| TEXAS INSTRUMENTS INCORPORATED
| Standard Linear and Logic Group
| IBIS Model of PCA9544A
| 4-CHANNEL I2C AND SMBus MULTIPLEXER WITH INTERRUPT LOGIC
| This file contains package information for the following:
|  TSSOP 20-pin (PW) package as [Component] PCA9544_PW
|  QFN 20-pin (RGY) package as [Component] PCA9544_RGY
|  SOIC 20-pin (DW) package as [Component] PCA9544_DW
|  TVSOP 20-pin (DGV) package as [Component] PCA9544_DGV
|  VFBGA 20-pin (GQN) package as [Component] PCA9544_GQN
|  VFBGA 20-pin (ZQN) package as [Component] PCA9544_ZQN
| This device can be powered at the following Vccs:
|  5 volt Vcc
|  3.3 volt Vcc
|  2.5 volt Vcc
| This file provides unique models under the [Model Selector] for each Vcc.
| For operation at a specific Vcc, select the appropriate model after each
| [Model Selector] keyword.
[IBIS Ver]   3.2
[Comment char]  |_char
[File Name]   pca9544a.ibs
[File Rev]   1.1 | a_die
[Date]   February 12, 2007
[Source]   Data created from TI-SPICE simulations at TI-SLL.
[Notes]   The following is an IBIS list for the PCA9544A.
   Please contact sllibis@ti.com with questions and
   comments concerning SLL IBIS models.
   This IBIS model is created from a BA (back annotated netlist)
   - FILE REV HISTORY
   - 1.1 Release IBIS file on 2/13/07
   - Power clamp data has been deleted in all models except
   SDA terminator models as there is no power-clamp diode.
   - Non-monotonic data due to FET characteristics.
[Disclaimer] Property of Texas Instruments Incorporated.  Unauthorized
   reproduction and/or distribution is strictly prohibited.
   This product is protected under copyright law.
   Created  2007, (C) Copyright  2007, Texas Instruments
   Incorporated, All Rights Reserved
   UNLESS THERE IS A SIGNED, WRITTEN AGREEMENT TO THE
   CONTRARY, TEXAS INSTRUMENTS (TI) IS PROVIDING THE IBIS
   MODELS  AND WITHOUT ANY WARRANTY, EXPRESSED OR
   IMPLIED.  TI assumes no liability for:
   1) the accuracy of the IBIS models provided to your
   company;
   2) the proper functioning of these IBIS Models in your
   design or for any resulting applications; or
   3) infringement of patents, copyrights or intellectual
   property rights resulting from your use of these IBIS
   models.
   TI provides IBIS Models as a service to our customers.
   You and your company shall not distribute, sell or give
   these models to anyone else without prior written
   permission from TI.
   TI reserves the right to make changes to our products or
   to discontinue any semiconductor product or service
   without notice, and advises our customers to obtain the
   latest version of relevant information to verify, before
   placing orders, that the information being relied on is
   current.
   Please be aware that your receipt and use of the IBIS
   information provided shall serve as acceptance of these
   terms and conditions.  If you do not accept these terms,
   you should return or destroy the IBIS models and any
   other accompanying information immediately.
| Component PCA9544A_PW 20-PIN TSSOP
[Component]   PCA9544A_PW
[Manufacturer]   Texas Instruments, Inc.
[Package]
|   typ   min   max
R_pkg   5.000e-02   4.200e-02   6.000e-02
L_pkg   2.802e-09   2.248e-09   3.553e-09
C_pkg   3.170e-13   2.020e-13   4.430e-13
[Pin]   signal_name   model_name   R_pin   L_pin   C_pin
1   A0   PCA9544_A   5.500e-02   3.461e-09   4.400e-13
2   A1   PCA9544_A   5.500e-02   3.150e-09   4.010e-13
3   A2   PCA9544_A   4.200e-02   2.619e-09   3.020e-13
4   NINT0   PCA9544_INTX   4.500e-02   2.273e-09   2.020e-13
5   SD0   PCA9544_SDX   4.500e-02   2.248e-09   2.240e-13
6   SC0   PCA9544_SCX   4.500e-02   2.273e-09   2.260e-13
7   NINT1   PCA9544_INTX   4.400e-02   2.323e-09   2.050e-13
8   SD1   PCA9544_SDX   4.600e-02   2.704e-09   3.070e-13
9   SC1   PCA9544_SCX   6.000e-02   3.265e-09   4.110e-13
10   GND   GND   5.700e-02   3.506e-09   4.360e-13
11   NINT2   PCA9544_INTX   5.800e-02   3.553e-09   4.370e-13
12   SD2   PCA9544_SDX   5.800e-02   3.193e-09   4.050e-13
13   SC2   PCA9544_SCX   4.200e-02   2.704e-09   3.110e-13
14   NINT3   PCA9544_INTX   4.600e-02   2.392e-09   2.100e-13
15   SD3   PCA9544_SDX   4.700e-02   2.334e-09   2.290e-13
16   SC3   PCA9544_SCX   4.700e-02   2.300e-09   2.270e-13
17   NINT   PCA9544_INT   4.700e-02   2.349e-09   2.070e-13
18   SCL   PCA9544_SCL   4.500e-02   2.677e-09   3.060e-13
19   SDA   PCA9544_SDA   6.000e-02   3.235e-09   4.060e-13
20   VCC   POWER   5.600e-02   3.487e-09   4.430e-13
| Component PCA9544A_RGY 20-PIN QFN
[Component]   PCA9544A_RGY
[Manufacturer]   Texas Instruments, Inc.
[Package]
|   typ   min   max
R_pkg   5.000e-02   4.600e-02   5.500e-02
L_pkg   1.119e-09   1.025e-09   1.227e-09
C_pkg   3.520e-13   3.440e-13   3.630e-13
[Pin]   signal_name   model_name   R_pin   L_pin   C_pin
1   A0   PCA9544_A   5.200e-02   1.167e-09   3.600e-13
2   A1   PCA9544_A   4.700e-02   1.049e-09   3.440e-13
3   A2   PCA9544_A   4.700e-02   1.055e-09   3.450e-13
4   NINT0   PCA9544_INTX   5.000e-02   1.119e-09   3.500e-13
5   SD0   PCA9544_SDX   5.500e-02   1.227e-09   3.600e-13
6   SC0   PCA9544_SCX   5.200e-02   1.167e-09   3.550e-13
7   NINT1   PCA9544_INTX   4.900e-02   1.087e-09   3.480e-13
8   SD1   PCA9544_SDX   4.700e-02   1.054e-09   3.460e-13
9   SC1   PCA9544_SCX   4.900e-02   1.091e-09   3.490e-13
10   GND   GND   5.300e-02   1.184e-09   3.620e-13
11   NINT2   PCA9544_INTX   5.300e-02   1.181e-09   3.600e-13
12   SD2   PCA9544_SDX   5.000e-02   1.108e-09   3.490e-13
13   SC2   PCA9544_SCX   4.800e-02   1.075e-09   3.470e-13
14   NINT3   PCA9544_INTX   5.000e-02   1.107e-09   3.490e-13
15   SD3   PCA9544_SDX   5.400e-02   1.200e-09   3.620e-13
16   SC3   PCA9544_SCX   5.100e-02   1.141e-09   3.570e-13
17   NINT   PCA9544_INT   4.700e-02   1.043e-09   3.440e-13
18   SCL   PCA9544_SCL   4.600e-02   1.025e-09   3.440e-13
19   SDA   PCA9544_SDA   4.900e-02   1.090e-09   3.490e-13
20   VCC   POWER   5.400e-02   1.204e-09   3.630e-13
| Component PCA9544A_DW 20-PIN SOIC
[Component]   PCA9544A_DW
[Manufacturer]   Texas Instruments, Inc.
[Package]
|   typ   min   max
R_pkg   3.800e-02   3.300e-02   4.500e-02
L_pkg   5.012e-09   4.110e-09   6.349e-09
C_pkg   7.170e-13   5.300e-13   8.680e-13
[Pin]   signal_name   model_name   R_pin   L_pin   C_pin
1   A0   PCA9544_A   4.200e-02   6.336e-09   8.650e-13
2   A1   PCA9544_A   4.300e-02   5.542e-09   8.670e-13
3   A2   PCA9544_A   3.400e-02   4.714e-09   7.320e-13
4   NINT0   PCA9544_INTX   3.400e-02   4.377e-09   5.910e-13
5   SD0   PCA9544_SDX   3.600e-02   4.130e-09   5.330e-13
6   SC0   PCA9544_SCX   3.500e-02   4.111e-09   5.300e-13
7   NINT1   PCA9544_INTX   3.400e-02   4.284e-09   5.830e-13
8   SD1   PCA9544_SDX   3.400e-02   4.634e-09   7.260e-13
9   SC1   PCA9544_SCX   4.000e-02   5.518e-09   8.650e-13
10   GND   GND   4.300e-02   6.349e-09   8.660e-13
11   NINT2   PCA9544_INTX   4.100e-02   6.281e-09   8.610e-13
12   SD2   PCA9544_SDX   4.500e-02   5.561e-09   8.680e-13
13   SC2   PCA9544_SCX   3.300e-02   4.778e-09   7.420e-13
14   NINT3   PCA9544_INTX   3.500e-02   4.414e-09   5.960e-13
15   SD3   PCA9544_SDX   3.500e-02   4.110e-09   5.330e-13
16   SC3   PCA9544_SCX   3.600e-02   4.130e-09   5.330e-13
17   NINT   PCA9544_INT   3.400e-02   4.377e-09   5.910e-13
18   SCL   PCA9544_SCL   3.400e-02   4.714e-09   7.310e-13
19   SDA   PCA9544_SDA   4.300e-02   5.569e-09   8.680e-13
20   VCC   POWER   4.200e-02   6.308e-09   8.640e-13
| Component PCA9544A_DGV 20-PIN TVSOP
[Component]   PCA9544A_DGV
[Manufacturer]   Texas Instruments, Inc.
[Package]
|   typ   min   max
R_pkg   4.400e-02   3.800e-02   4.800e-02
L_pkg   2.561e-09   2.236e-09   2.961e-09
C_pkg   3.420e-13   2.640e-13   4.460e-13
[Pin]   signal_name   model_name   R_pin   L_pin   C_pin
1   A0   PCA9544_A   4.400e-02   2.935e-09   4.170e-13
2   A1   PCA9544_A   4.200e-02   2.869e-09   4.460e-13
3   A2   PCA9544_A   4.300e-02   2.399e-09   3.160e-13
4   NINT0   PCA9544_INTX   4.400e-02   2.236e-09   2.650e-13
5   SD0   PCA9544_SDX   4.600e-02   2.278e-09   2.640e-13
6   SC0   PCA9544_SCX   4.500e-02   2.274e-09   2.640e-13
7   NINT1   PCA9544_INTX   4.400e-02   2.285e-09   2.690e-13
8   SD1   PCA9544_SDX   4.300e-02   2.452e-09   3.200e-13
9   SC1   PCA9544_SCX   4.400e-02   2.900e-09   4.460e-13
10   GND   GND   4.400e-02   2.961e-09   4.180e-13
11   NINT2   PCA9544_INTX   4.500e-02   2.954e-09   4.180e-13
12   SD2   PCA9544_SDX   4.200e-02   2.847e-09   4.430e-13
13   SC2   PCA9544_SCX   4.500e-02   2.453e-09   3.190e-13
14   NINT3   PCA9544_INTX   4.500e-02   2.297e-09   2.690e-13
15   SD3   PCA9544_SDX   4.800e-02   2.334e-09   2.680e-13
16   SC3   PCA9544_SCX   4.800e-02   2.335e-09   2.670e-13
17   NINT   PCA9544_INT   4.600e-02   2.299e-09   2.680e-13
18   SCL   PCA9544_SCL   4.600e-02   2.457e-09   3.200e-13
19   SDA   PCA9544_SDA   4.300e-02   2.848e-09   4.410e-13
20   VCC   POWER   3.800e-02   2.812e-09   4.080e-13
| Component PCA9544A_GQN 20-PIN VFBGA
[Component]   PCA9544A_GQN
[Manufacturer]   Texas Instruments, Inc.
[Package]
|   typ   min   max
R_pkg   4.300e-02   3.300e-02   6.100e-02
L_pkg   1.317e-09   8.960e-10   2.088e-09
C_pkg   1.130e-13   6.400e-14   1.900e-13
[Pin]   signal_name   model_name   R_pin   L_pin   C_pin
1   A0   PCA9544_A   3.800e-02   1.199e-09   1.210e-13
2   A1   PCA9544_A   4.000e-02   1.067e-09   1.020e-13
3   A2   PCA9544_A   6.100e-02   1.999e-09   1.900e-13
4   NINT0   PCA9544_INTX   3.300e-02   9.630e-10   7.100e-14
5   SD0   PCA9544_SDX   4.900e-02   1.523e-09   1.230e-13
6   SC0   PCA9544_SCX   3.300e-02   8.960e-10   6.400e-14
7   NINT1   PCA9544_INTX   6.100e-02   1.899e-09   1.640e-13
8   SD1   PCA9544_SDX   3.300e-02   8.980e-10   6.700e-14
9   SC1   PCA9544_SCX   4.900e-02   1.514e-09   1.280e-13
10   GND   GND   3.600e-02   1.006e-09   9.400e-14
11   NINT2   PCA9544_INTX   4.900e-02   1.683e-09   1.460e-13
12   SD2   PCA9544_SDX   3.300e-02   1.121e-09   8.900e-14
13   SC2   PCA9544_SCX   6.100e-02   2.088e-09   1.730e-13
14   NINT3   PCA9544_INTX   3.300e-02   1.027e-09   7.100e-14
15   SD3   PCA9544_SDX   4.900e-02   1.558e-09   1.240e-13
16   SC3   PCA9544_SCX   3.300e-02   9.280e-10   6.700e-14
17   NINT   PCA9544_INT   6.100e-02   1.921e-09   1.770e-13
18   SCL   PCA9544_SCL   3.300e-02   9.010e-10   7.700e-14
19   SDA   PCA9544_SDA   3.700e-02   9.900e-10   9.800e-14
20   VCC   POWER   3.500e-02   1.168e-09   1.190e-13
| Component PCA9544A_ZQN 20-PIN VFBGA
[Component]   PCA9544A_ZQN
[Manufacturer]   Texas Instruments, Inc.
[Package]
|   typ   min   max
R_pkg   4.300e-02   3.300e-02   6.100e-02
L_pkg   1.317e-09   8.960e-10   2.088e-09
C_pkg   1.130e-13   6.400e-14   1.900e-13
[Pin]   signal_name   model_name   R_pin   L_pin   C_pin
1   A0   PCA9544_A   3.800e-02   1.199e-09   1.210e-13
2   A1   PCA9544_A   4.000e-02   1.067e-09   1.020e-13
3   A2   PCA9544_A   6.100e-02   1.999e-09   1.900e-13
4   NINT0   PCA9544_INTX   3.300e-02   9.630e-10   7.100e-14
5   SD0   PCA9544_SDX   4.900e-02   1.523e-09   1.230e-13
6   SC0   PCA9544_SCX   3.300e-02   8.960e-10   6.400e-14
7   NINT1   PCA9544_INTX   6.100e-02   1.899e-09   1.640e-13
8   SD1   PCA9544_SDX   3.300e-02   8.980e-10   6.700e-14
9   SC1   PCA9544_SCX   4.900e-02   1.514e-09   1.280e-13
10   GND   GND   3.600e-02   1.006e-09   9.400e-14
11   NINT2   PCA9544_INTX   4.900e-02   1.683e-09   1.460e-13
12   SD2   PCA9544_SDX   3.300e-02   1.121e-09   8.900e-14
13   SC2   PCA9544_SCX   6.100e-02   2.088e-09   1.730e-13
14   NINT3   PCA9544_INTX   3.300e-02   1.027e-09   7.100e-14
15   SD3   PCA9544_SDX   4.900e-02   1.558e-09   1.240e-13
16   SC3   PCA9544_SCX   3.300e-02   9.280e-10   6.700e-14
17   NINT   PCA9544_INT   6.100e-02   1.921e-09   1.770e-13
18   SCL   PCA9544_SCL   3.300e-02   9.010e-10   7.700e-14
19   SDA   PCA9544_SDA   3.700e-02   9.900e-10   9.800e-14
20   VCC   POWER   3.500e-02   1.168e-09   1.190e-13
[Series Switch Groups]
| Function Group States
On  1 /   | SDA/SCL<->SD/SC0
On  2 /   | SDA/SCL<->SD/SC1
On  3 /   | SDA/SCL<->SD/SC2
On  4 /   | SDA/SCL<->SD/SC3
[Series Pin Mapping]   pin_2   model_name   function_table_group
5   19   PCA9544_SDX_50_S   1
| 5   19   PCA9544_SDX_33_S   1
| 5   19   PCA9544_SDX_25_S   1
19   5   PCA9544_SDA_50_S   1
| 19   5   PCA9544_SDA_33_S   1
| 19   5   PCA9544_SDA_25_S   1
6   18   PCA9544_SCX_50_S   1
| 6   18   PCA9544_SCX_33_S   1
| 6   18   PCA9544_SCX_25_S   1
18   6   PCA9544_SCL_50_S   1
| 18   6   PCA9544_SCL_33_S   1
| 18   6   PCA9544_SCL_25_S   1
8   19   PCA9544_SDX_50_S   2
| 8   19   PCA9544_SDX_33_S   2
| 8   19   PCA9544_SDX_25_S   2
19   8   PCA9544_SDA_50_S   2
| 19   8   PCA9544_SDA_33_S   2
| 19   8   PCA9544_SDA_25_S   2
9   18   PCA9544_SCX_50_S   2
| 9   18   PCA9544_SCX_33_S   2
| 9   18   PCA9544_SCX_25_S   2
18   9   PCA9544_SCL_50_S   2
| 18   9   PCA9544_SCL_33_S   2
| 18   9   PCA9544_SCL_25_S   2
12   19   PCA9544_SDX_50_S   3
| 12   19   PCA9544_SDX_33_S   3
| 12   19   PCA9544_SDX_25_S   3
19   12   PCA9544_SDA_50_S   3
| 19   12   PCA9544_SDA_33_S   3
| 19   12   PCA9544_SDA_25_S   3
13   18   PCA9544_SCX_50_S   3
| 13   18   PCA9544_SCX_33_S   3
| 13   18   PCA9544_SCX_25_S   3
18   13   PCA9544_SCL_50_S   3
| 18   13   PCA9544_SCL_33_S   3
| 18   13   PCA9544_SCL_25_S   3
15   19   PCA9544_SDX_50_S   4
| 15   19   PCA9544_SDX_33_S   4
| 15   19   PCA9544_SDX_25_S   4
19   15   PCA9544_SDA_50_S   4
| 19   15   PCA9544_SDA_33_S   4
| 19   15   PCA9544_SDA_25_S   4
16   18   PCA9544_SCX_50_S   4
| 16   18   PCA9544_SCX_33_S   4
| 16   18   PCA9544_SCX_25_S   4
18   16   PCA9544_SCL_50_S   4
| 18   16   PCA9544_SCL_33_S   4
| 18   16   PCA9544_SCL_25_S   4
| Model PCA9544_INTX
[Model Selector]   PCA9544_INTX
PCA9544_INTX_50   5 volt Vcc
PCA9544_INTX_33   3.3 volt Vcc
PCA9544_INTX_25   2.5 volt Vcc
| Model PCA9544_A
[Model Selector]   PCA9544_A
PCA9544_A_50   5 volt Vcc
PCA9544_A_33   3.3 volt Vcc
PCA9544_A_25   2.5 volt Vcc
| Model PCA9544_INT
[Model Selector]   PCA9544_INT
PCA9544_INT_50   5 volt Vcc
PCA9544_INT_33   3.3 volt Vcc
PCA9544_INT_25   2.5 volt Vcc
| Model PCA9544_SDX
[Model Selector]   PCA9544_SDX
PCA9544_SDX_50   5 volt Vcc
PCA9544_SDX_33   3.3 volt Vcc
PCA9544_SDX_25   2.5 volt Vcc
| Model PCA9544_SDX_S
[Model Selector]   PCA9544_SDX_S
PCA9544_SDX_50_S   5 volt Vcc
PCA9544_SDX_33_S   3.3 volt Vcc
PCA9544_SDX_25_S   2.5 volt Vcc
| Model PCA9544_SCX
[Model Selector]   PCA9544_SCX
PCA9544_SCX_50   5 volt Vcc
PCA9544_SCX_33   3.3 volt Vcc
PCA9544_SCX_25   2.5 volt Vcc
| Model PCA9544_SCX_S
[Model Selector]   PCA9544_SCX_S
PCA9544_SCX_50_S   5 volt Vcc
PCA9544_SCX_33_S   3.3 volt Vcc
PCA9544_SCX_25_S   2.5 volt Vcc
| Model PCA9544_SCL
[Model Selector]   PCA9544_SCL
PCA9544_SCL_50   5 volt Vcc
PCA9544_SCL_33   3.3 volt Vcc
PCA9544_SCL_25   2.5 volt Vcc
| Model PCA9544_SCL_S
[Model Selector]   PCA9544_SCL_S
PCA9544_SCL_50_S   5 volt Vcc
PCA9544_SCL_33_S   3.3 volt Vcc
PCA9544_SCL_25_S   2.5 volt Vcc
| Model PCA9544_SDA
[Model Selector]   PCA9544_SDA
PCA9544_SDA_50   5 volt Vcc
PCA9544_SDA_33   3.3 volt Vcc
PCA9544_SDA_25   2.5 volt Vcc
| Model PCA9544_SDA_S
[Model Selector]   PCA9544_SDA_S
PCA9544_SDA_50_S   5 volt Vcc
PCA9544_SDA_33_S   3.3 volt Vcc
PCA9544_SDA_25_S   2.5 volt Vcc
[Model]   PCA9544_SDX_50_S
Model_type  Series_switch
| variable   typ   min   max
C_comp   0   0   0
[Temperature Range]   40   100   -40
| Ambient temperature   25   85   -40
[Voltage range]   5   4.5   5.5
[On]
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[Off]
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[Model]   PCA9544_SDX_33_S
Model_type  Series_switch
| variable   typ   min   max
C_comp   0   0   0
[Temperature Range]   40   100   -40
| Ambient temperature   25   85   -40
[Voltage range]   3.3   3   3.6
[On]
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[Off]
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[Model]   PCA9544_SDX_25_S
Model_type  Series_switch
| variable   typ   min   max
C_comp   0   0   0
[Temperature Range]   40   100   -40
| Ambient temperature   25   85   -40
[Voltage range]   2.5   2.3   2.7
[On]
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[Off]
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[Model]   PCA9544_SCX_50_S
Model_type  Series_switch
| variable   typ   min   max
C_comp   0   0   0
[Temperature Range]   40   100   -40
| Ambient temperature   25   85   -40
[Voltage range]   5   4.5   5.5
[On]
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[Off]
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[Model]   PCA9544_SCX_33_S
Model_type  Series_switch
| variable   typ   min   max
C_comp   0   0   0
[Temperature Range]   40   100   -40
| Ambient temperature   25   85   -40
[Voltage range]   3.3   3   3.6
[On]
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[Off]
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[Model]   PCA9544_SCX_25_S
Model_type  Series_switch
| variable   typ   min   max
C_comp   0   0   0
[Temperature Range]   40   100   -40
| Ambient temperature   25   85   -40
[Voltage range]   2.5   2.3   2.7
[On]
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[Off]
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[Model]   PCA9544_SCL_50_S
Model_type  Series_switch
| variable   typ   min   max
C_comp   0   0   0
[Temperature Range]   40   100   -40
| Ambient temperature   25   85   -40
[Voltage range]   5   4.5   5.5
[On]
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[Off]
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[Model]   PCA9544_SCL_33_S
Model_type  Series_switch
| variable   typ   min   max
C_comp   0   0   0
[Temperature Range]   40   100   -40
| Ambient temperature   25   85   -40
[Voltage range]   3.3   3   3.6
[On]
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[Off]
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[Model]   PCA9544_SCL_25_S
Model_type  Series_switch
| variable   typ   min   max
C_comp   0   0   0
[Temperature Range]   40   100   -40
| Ambient temperature   25   85   -40
[Voltage range]   2.5   2.3   2.7
[On]
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[Off]
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[Model]   PCA9544_SDA_50_S
Model_type  Series_switch
| variable   typ   min   max
C_comp   0   0   0
[Temperature Range]   40   100   -40
| Ambient temperature   25   85   -40
[Voltage range]   5   4.5   5.5
[On]
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[Off]
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[Model]   PCA9544_SDA_33_S
Model_type  Series_switch
| variable   typ   min   max
C_comp   0   0   0
[Temperature Range]   40   100   -40
| Ambient temperature   25   85   -40
[Voltage range]   3.3   3   3.6
[On]
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[Off]
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[Model]   PCA9544_SDA_25_S
Model_type  Series_switch
| variable   typ   min   max
C_comp   0   0   0
[Temperature Range]   40   100   -40
| Ambient temperature   25   85   -40
[Voltage range]   2.5   2.3   2.7
[On]
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[Off]
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| Models and submodels in the file (33): PCA9544_INTX_50 (Input), PCA9544_INTX_33 (Input), PCA9544_INTX_25 (Input), PCA9544_A_50 (Input), PCA9544_A_33 (Input), PCA9544_A_25 (Input), PCA9544_INT_50 (Open_drain), PCA9544_INT_33 (Open_drain), PCA9544_INT_25 (Open_drain), PCA9544_SDX_50_S (Series_switch), PCA9544_SDX_50 (Terminator), PCA9544_SDX_33_S (Series_switch), PCA9544_SDX_33 (Terminator), PCA9544_SDX_25_S (Series_switch), PCA9544_SDX_25 (Terminator), PCA9544_SCX_50_S (Series_switch), PCA9544_SCX_50 (Terminator), PCA9544_SCX_33_S (Series_switch), PCA9544_SCX_33 (Terminator), PCA9544_SCX_25_S (Series_switch), PCA9544_SCX_25 (Terminator), PCA9544_SCL_50_S (Series_switch), PCA9544_SCL_50 (Terminator), PCA9544_SCL_33_S (Series_switch), PCA9544_SCL_33 (Terminator), PCA9544_SCL_25_S (Series_switch), PCA9544_SCL_25 (Terminator), PCA9544_SDA_50_S (Series_switch), PCA9544_SDA_50 (Terminator), PCA9544_SDA_33_S (Series_switch), PCA9544_SDA_33 (Terminator), PCA9544_SDA_25_S (Series_switch), PCA9544_SDA_25 (Terminator)
